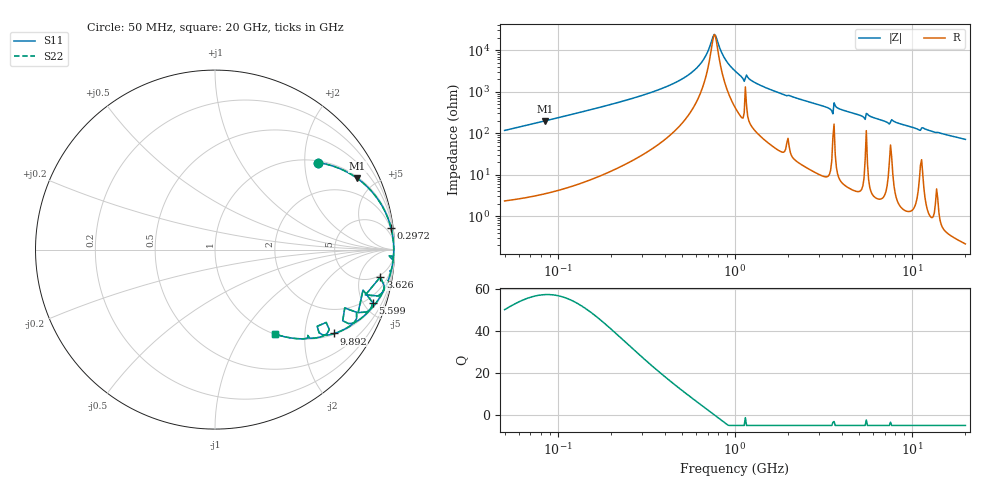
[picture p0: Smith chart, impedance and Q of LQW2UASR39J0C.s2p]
!Murata Part Number: LQW2UASR39J0C
!These Parameters are Measured in Series Mode Connection
!  o--[Z]--o
!Port1  Port2
!  o-------o
!Freq. Start=50[MHz] Stop=20[GHz], 401[Steps]
# Hz S RI R 50
!Freq.(Hz) S11(Real) S11(Imag) S21(Real) S21(Imag) S12(Real) S12(Imag) S22(Real) S22(Imag)
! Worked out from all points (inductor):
!   401 points, 50 MHz to 20 GHz, reference 50 ohm
!   read as one part in series: L = 368 nH near 51.52 MHz
!   highest Q = 57.2 at 84.46 MHz (marker M1), where L = 373 nH
!   self-resonance near 763.7 MHz
!   S11 on the Smith chart (normalised r, x): 50 MHz: 1.05, +2.33; 297.2 MHz: 2, +16; 3.626 GHz: 4, -10; 5.599 GHz: 1.37, -5.79; 9.892 GHz: 1.03, -2.83; 20 GHz: 1.00, -1.42
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5e7  0.5737 0.4847  0.4263 -0.4847  0.4263 -0.4847  0.5737 0.4847
8.445984e7  0.7923 0.397  0.2077 -0.397  0.2077 -0.397  0.7923 0.397
1.364002e8  0.9094 0.2776  0.0906 -0.2776  0.0906 -0.2776  0.9094 0.2776
2.972233e8  0.9807 0.1208  0.0193 -0.1208  0.0193 -0.1208  0.9807 0.1208
3.721004e8  0.9879 0.0875  0.0121 -0.0875  0.0121 -0.0875  0.9879 0.0875
6.009314e8  0.9951 0.0275  0.00493 -0.0275  0.00493 -0.0275  0.9951 0.0275
6.774326e8  0.9957 0.0139  0.00434 -0.0139  0.00434 -0.0139  0.9957 0.0139
7.636728e8  0.9959 0.000345  0.00414 -0.000345  0.00414 -0.000345  0.9959 0.000345
7.868965e8  0.9959 -0.00304  0.00414 0.00304  0.00414 0.00304  0.9959 -0.00304
8.738837e8  0.9956 -0.015  0.00436 0.015  0.00436 0.015  0.9956 -0.015
1e9  0.9949 -0.031  0.00514 0.031  0.00514 0.031  0.9949 -0.031
1.094034e9  0.9933 -0.0441  0.00666 0.0441  0.00666 0.0441  0.9933 -0.0441
1.179116e9  0.9929 -0.0439  0.00707 0.0439  0.00707 0.0439  0.9929 -0.0439
1.498439e9  0.9895 -0.0794  0.0105 0.0794  0.0105 0.0794  0.9895 -0.0794
2.728004e9  0.9629 -0.1778  0.0371 0.1778  0.0371 0.1778  0.9629 -0.1778
3.466789e9  0.9257 -0.2457  0.0743 0.2457  0.0743 0.2457  0.9257 -0.2457
3.626126e9  0.9211 -0.1534  0.0789 0.1534  0.0789 0.1534  0.9211 -0.1534
5.273168e9  0.8574 -0.3391  0.1426 0.3391  0.1426 0.3391  0.8574 -0.3391
5.598765e9  0.8789 -0.2958  0.1211 0.2958  0.1211 0.2958  0.8789 -0.2958
7.442007e9  0.7117 -0.3964  0.2883 0.3964  0.2883 0.3964  0.7117 -0.3964
9.892087e9  0.6647 -0.4674  0.3353 0.4674  0.3353 0.4674  0.6647 -0.4674
2e10  0.3351 -0.4705  0.6649 0.4705  0.6649 0.4705  0.3351 -0.4705
